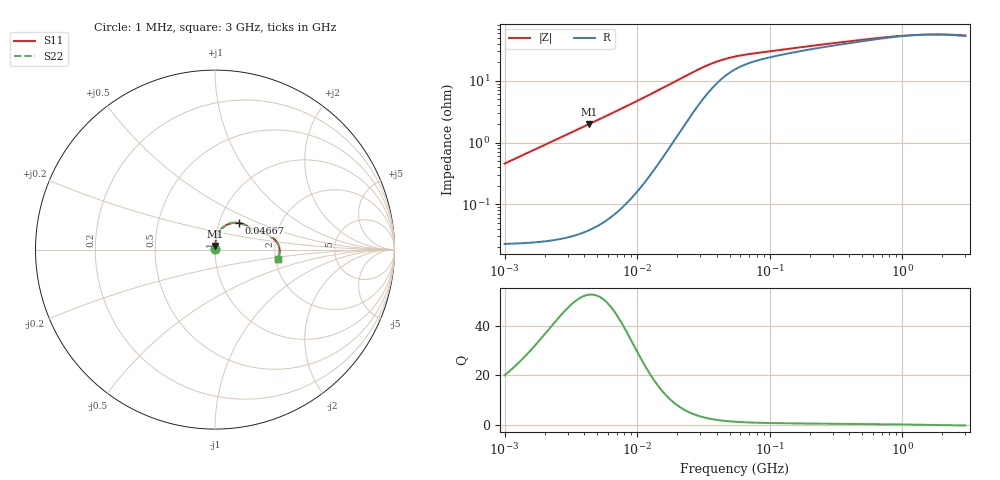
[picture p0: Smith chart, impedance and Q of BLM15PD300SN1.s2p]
! BLM15PD300SN1
# Hz S RI R 50
!Freq.(Hz) S11(Real) S11(Imag) S21(Real) S21(Imag) S12(Real) S12(Imag) S22(Real) S22(Imag)
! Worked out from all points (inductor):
!   401 points, 1 MHz to 3 GHz, reference 50 ohm
!   read as one part in series: L = 72.4 nH near 1.041 MHz
!   highest Q = 52.5 at 4.311 MHz (marker M1), where L = 72.9 nH
!   self-resonance near 1.64 GHz
!   S11 on the Smith chart (normalised r, x): 1 MHz: 1.00, +0.01; 46.67 MHz: 1.24, +0.38; 3 GHz: 2.06, -0.24
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1000000  0.000248 0.00454  0.9998 -0.00454  0.9998 -0.00454  0.000248 0.00454
1040844  0.00025 0.00473  0.9997 -0.00473  0.9997 -0.00473  0.00025 0.00473
3823119  0.000644 0.0175  0.9994 -0.0175  0.9994 -0.0175  0.000644 0.0175
4310966  0.000765 0.0197  0.9992 -0.0197  0.9992 -0.0197  0.000765 0.0197
8513927  0.00266 0.0396  0.9973 -0.0396  0.9973 -0.0396  0.00266 0.0396
1.461624e7  0.00959 0.0701  0.9904 -0.0701  0.9904 -0.0701  0.00959 0.0701
2.137957e7  0.0265 0.1037  0.9735 -0.1037  0.9735 -0.1037  0.0265 0.1037
2.559965e7  0.0425 0.1219  0.9575 -0.1219  0.9575 -0.1219  0.0425 0.1219
2.944989e7  0.0598 0.1348  0.9402 -0.1348  0.9402 -0.1348  0.0598 0.1348
3.320783e7  0.0778 0.1434  0.9222 -0.1434  0.9222 -0.1434  0.0778 0.1434
3.74453e7  0.0977 0.1486  0.9023 -0.1486  0.9023 -0.1486  0.0977 0.1486
4.138676e7  0.1146 0.1499  0.8854 -0.1499  0.8854 -0.1499  0.1146 0.1499
4.666789e7  0.134 0.1482  0.866 -0.1482  0.866 -0.1482  0.134 0.1482
5.477226e7  0.1565 0.142  0.8435 -0.142  0.8435 -0.142  0.1565 0.142
8.173662e7  0.1956 0.1225  0.8044 -0.1225  0.8044 -0.1225  0.1956 0.1225
2.094008e8  0.2588 0.0955  0.7412 -0.0955  0.7412 -0.0955  0.2588 0.0955
4.853736e8  0.3098 0.0724  0.6902 -0.0724  0.6902 -0.0724  0.3098 0.0724
8.005644e8  0.3383 0.0501  0.6617 -0.0501  0.6617 -0.0501  0.3383 0.0501
1.125055e9  0.3525 0.0284  0.6475 -0.0284  0.6475 -0.0284  0.3525 0.0284
1.581072e9  0.3596 0.00289  0.6404 -0.00289  0.6404 -0.00289  0.3596 0.00289
2.177892e9  0.3589 -0.0233  0.6411 0.0233  0.6411 0.0233  0.3589 -0.0233
3e9  0.3501 -0.0503  0.6499 0.0503  0.6499 0.0503  0.3501 -0.0503
